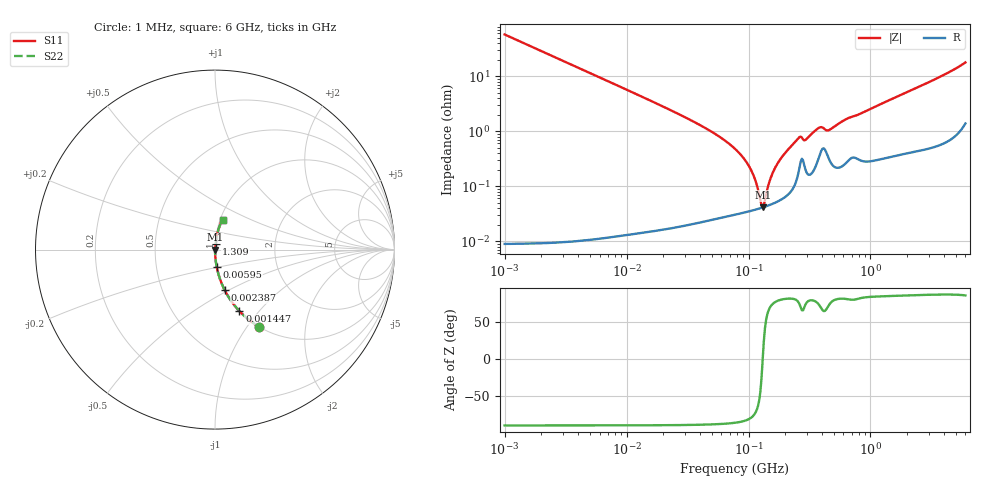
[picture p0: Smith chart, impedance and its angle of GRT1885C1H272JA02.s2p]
!Murata Part Number: GRT1885C1H272JA02
!These Parameters are Measured in Series Mode Connection
!Data Generated on Jun 19, 2026
!  o--ll--o
!Port1  Port2
!  o------o
!Operation Temp=25[degC], DC Bias Voltage=0[V]
!Freq. Start=1000[kHz] Stop=6[GHz] 401[Steps]
# Hz S RI R 50
!Freq.(Hz) S11(Real) S11(Imag) S21(Real) S21(Imag) S12(Real) S12(Imag) S22(Real) S22(Imag)
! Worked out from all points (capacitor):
!   401 points, 1 MHz to 6 GHz, reference 50 ohm
!   read as one part in series: C = 2.78 nF near 1.044 MHz
!   lowest |Z| = 41.1 mohm at 130.5 MHz (marker M1)
!   series resonance near 130.7 MHz, so ESL is about 530 pH
!   S11 on the Smith chart (normalised r, x): 1 MHz: 1.00, -1.15; 1.447 MHz: 1.00, -0.79; 2.387 MHz: 1.00, -0.48; 5.95 MHz: 1.00, -0.19; 1.309 GHz: 1.01, +0.07; 6 GHz: 1.03, +0.35
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1000000  0.2473 -0.4314  0.7527 0.4314  0.7527 0.4314  0.2473 -0.4314
1447343  0.1356 -0.3423  0.8644 0.3423  0.8644 0.3423  0.1356 -0.3423
2386795  0.0546 -0.2269  0.9454 0.2269  0.9454 0.2269  0.0546 -0.2269
4293785  0.0176 -0.131  0.9824 0.131  0.9824 0.131  0.0176 -0.131
5950055  0.00926 -0.0952  0.9907 0.0952  0.9907 0.0952  0.00926 -0.0952
1.843659e7  0.00108 -0.0304  0.9989 0.0304  0.9989 0.0304  0.00108 -0.0304
4.596069e7  0.000352 -0.0109  0.9996 0.0109  0.9996 0.0109  0.000352 -0.0109
7.745967e7  0.000326 -0.00477  0.9997 0.00477  0.9997 0.00477  0.000326 -0.00477
1.050294e8  0.000361 -0.00193  0.9996 0.00193  0.9996 0.00193  0.000361 -0.00193
1.249896e8  0.000398 -0.000394  0.9996 0.000394  0.9996 0.000394  0.000398 -0.000394
1.305463e8  0.000411 -1.22e-05  0.9996 1.22e-05  0.9996 1.22e-05  0.000411 -1.22e-05
1.363501e8  0.000424 0.000371  0.9996 -0.000371  0.9996 -0.000371  0.000424 0.000371
1.553559e8  0.000475 0.00154  0.9995 -0.00154  0.9995 -0.00154  0.000475 0.00154
1.848803e8  0.00058 0.00318  0.9994 -0.00318  0.9994 -0.00318  0.00058 0.00318
2.561955e8  0.00178 0.00724  0.9982 -0.00724  0.9982 -0.00724  0.00178 0.00724
2.919064e8  0.0021 0.00656  0.9979 -0.00656  0.9979 -0.00656  0.0021 0.00656
3.325952e8  0.00183 0.00894  0.9982 -0.00894  0.9982 -0.00894  0.00183 0.00894
3.872876e8  0.00406 0.011  0.9959 -0.011  0.9959 -0.011  0.00406 0.011
4.608893e8  0.00308 0.0101  0.9969 -0.0101  0.9969 -0.0101  0.00308 0.0101
1.309106e9  0.00432 0.0332  0.9957 -0.0332  0.9957 -0.0332  0.00432 0.0332
1.428092e9  0.00468 0.0363  0.9953 -0.0363  0.9953 -0.0363  0.00468 0.0363
6e9  0.0429 0.1675  0.9571 -0.1675  0.9571 -0.1675  0.0429 0.1675
